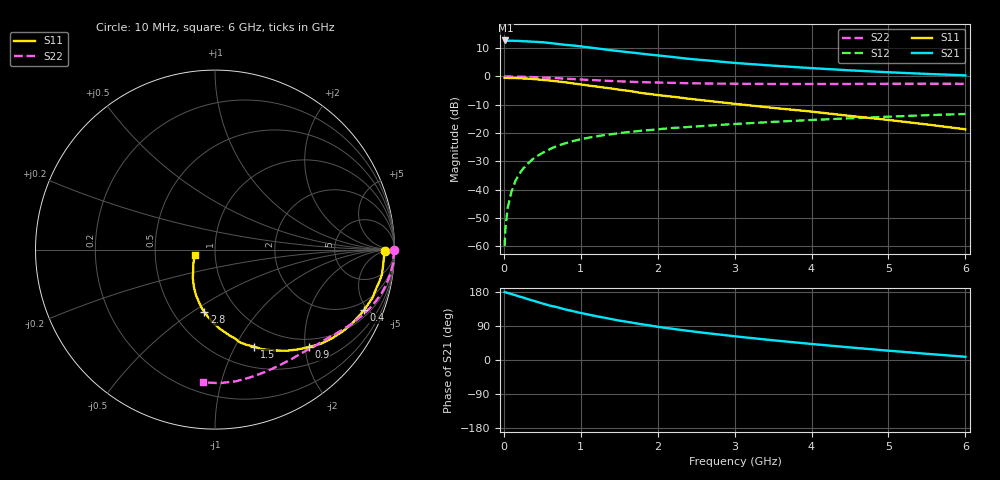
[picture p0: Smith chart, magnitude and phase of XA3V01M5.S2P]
! SIEMENS Discrete & RF Semiconductors
! BFY180
! Si NPN RF Bipolar Junction Transistor in MICRO-X
! VCE = 3 V  IC = 1.5 mA
! Common Emitter S-Parameters:  May  1997
# GHz  S  MA  R  50
!  f  S11  S21  S12  S22
! GHz  MAG  ANG  MAG  ANG  MAG  ANG  MAG  ANG
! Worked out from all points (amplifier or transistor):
!   36 points, 10 MHz to 6 GHz, reference 50 ohm
!   highest |S21| = 12.7 dB at 20 MHz (marker M1)
!   |S21| within 3 dB of that: start of sweep to 1.264 GHz
!   unconditionally stable (mu >= 1): 3.209 GHz to end of sweep
!   at 250 MHz: K = 0.10, MSG = 22.5 dB, |S12| = -32.6 dB
!   at 1.4 GHz: K = 0.61, MSG = 14.8 dB, |S12| = -20.4 dB
!   at 6 GHz: K = 1.07, MAG = 5.2 dB, |S12| = -13.3 dB
!   S11 on the Smith chart (normalised r, x): 10 MHz: 35, -6; 400 MHz: 1.37, -4.71; 900 MHz: 0.83, -2.08; 1.5 GHz: 0.73, -1.20; 2.8 GHz: 0.70, -0.56; 6 GHz: 0.80, -0.05
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0.01  0.9464 -0.5  4.295 179.3  0.001 87.7  0.9963 -0.2
0.02  0.945 -1.0  4.33 178.5  0.002 86.6  0.9999 -0.6
0.05  0.9421 -2.8  4.26 177.0  0.0048 85.7  0.9972 -1.5
0.1  0.9406 -5.8  4.294 174.0  0.0092 86.0  0.9938 -3.1
0.15  0.9401 -8.7  4.246 170.9  0.0142 85.3  0.9947 -4.6
0.25  0.9222 -14.2  4.196 164.8  0.0234 81.5  0.9889 -7.6
0.4  0.896 -22.2  4.102 155.4  0.037 75.7  0.9728 -11.8
0.5  0.8709 -27.6  4.034 149.3  0.0443 71.9  0.9597 -14.6
0.6  0.8466 -32.4  3.9 143.5  0.0521 68.9  0.9448 -17.1
0.8  0.7882 -41.8  3.618 133.3  0.0659 63.1  0.9146 -21.8
0.9  0.7534 -46.1  3.53 128.8  0.0722 60.6  0.8999 -24.0
1.1  0.6917 -54.5  3.268 119.9  0.0825 56.1  0.8697 -27.9
1.2  0.6642 -57.9  3.149 115.6  0.0873 53.8  0.8564 -29.8
1.5  0.5833 -68.0  2.805 104.0  0.0997 49.0  0.8205 -34.8
1.8  0.5067 -77.4  2.516 94.0  0.1101 45.5  0.7933 -39.2
2  0.4684 -82.5  2.357 87.6  0.1165 43.2  0.7807 -42.0
2.2  0.4381 -87.1  2.206 82.1  0.123 40.9  0.7705 -44.8
2.8  0.352 -99.8  1.835 67.2  0.139 36.3  0.7475 -52.4
3.5  0.2786 -112.0  1.552 52.0  0.1574 31.2  0.7377 -61.2
4.5  0.2007 -128.0  1.283 33.2  0.1822 24.1  0.7383 -74.1
5.5  0.1417 -148.1  1.109 16.3  0.2068 16.4  0.7445 -88.0
6  0.1164 -164.4  1.046 8.5  0.2173 12.3  0.7426 -95.0
